| IBIS file for GS81302xxxE
| Package: standard 165pin BGA
| DQ driver is programmable
| VDD 1.8V, VDDQ 1.5V or 1.8V
| Date:
| Rev 1.1 11/12/10 1) Pin F10 on Q36 pacakge changed from DIN to PROGBUF
[IBIS Ver]   4.2
[File name]   81302xxxe.ibs
[File Rev]   1.1
[Date]   11/12/10
[Component]   GS81302D08E
[Manufacturer]   GSI Technology
[Package]
|  variable   typ   min   max
R_pkg   0.2   0.1   0.5
L_pkg   3nH   1nH   5nH
C_pkg   1.5pF   1pF   3pF
[Package Model]   81302xxxE
[Pin Mapping] pulldown_ref pullup_ref gnd_clamp_ref power_clamp_ref ext_ref
|PIN   Pull-Down   Pull-Up   Power-clamp   Gnd-clamp   EXT-ref
 A1   VSS   VDDQ   VSS   VDD
 A2   NC   NC   VSS   VDD   VREF
 A3   NC   NC   VSS   VDD   VREF
 A4   NC   NC   VSS   VDD   VREF
 A5   NC   NC   VSS   VDD   VREF
 A6   NC   NC   VSS   VDD   VREF
 A7   NC   NC   VSS   VDD   VREF
 A8   NC   NC   VSS   VDD   VREF
 A9   NC   NC   VSS   VDD   VREF
 A10   NC   NC   VSS   VDD   VREF
 A11   VSS   VDDQ   VSS   VDD
 B1   NC   NC
 B2   NC   NC
 B3   NC   NC
 B4   NC   NC   VSS   VDD   VREF
 B5   NC   NC
 B6   NC   NC   VSS   VDD   VREF
 B7   NC   NC   VSS   VDD   VREF
 B8   NC   NC   VSS   VDD   VREF
 B9   NC   NC
 B10   NC   NC
 B11   VSS   VDDQ   VSS   VDD
 C1   NC   NC
 C2   NC   NC
 C3   NC   NC
 C4   VSS   NC
 C5   NC   NC   VSS   VDD   VREF
 C6   NC   NC
 C7   NC   NC   VSS   VDD   VREF
 C8   VSS   NC
 C9   NC   NC
 C10   NC   NC
 C11   NC   NC   VSS   VDD   VREF
 D1   NC   NC
 D2   NC   NC   VSS   VDD   VREF
 D3   NC   NC
 D4   VSS   NC
 D5   VSS   NC
 D6   VSS   NC
 D7   VSS   NC
 D8   VSS   NC
 D9   NC   NC
 D10   NC   NC
 D11   NC   NC
 E1   NC   NC
 E2   NC   NC
 E3   NC   NC
 E4   NC   VDDQ
 E5   VSS   NC
 E6   VSS   NC
 E7   VSS   NC
 E8   NC   VDDQ
 E9   NC   NC
 E10   NC   NC   VSS   VDD   VREF
 E11   VSS   VDDQ   VSS   VDD
 F1   NC   NC
 F2   NC   NC
 F3   NC   NC
 F4   NC   VDDQ
 F5   NC   VDD
 F6   VSS   NC
 F7   NC   VDD
 F8   NC   VDDQ
 F9   NC   NC
 F10   NC   NC
 F11   NC   NC
 G1   NC   NC
 G2   NC   NC   VSS   VDD   VREF
 G3   VSS   VDDQ   VSS   VDD
 G4   NC   VDDQ
 G5   NC   VDD
 G6   VSS   NC
 G7   NC   VDD
 G8   NC   VDDQ
 G9   NC   NC
 G10   NC   NC
 G11   NC   NC
 H1   NC   NC   VSS   VDD   VREF
 H2   NC   VREF
 H3   NC   VDDQ
 H4   NC   VDDQ
 H5   NC   VDD
 H6   VSS   NC
 H7   NC   VDD
 H8   NC   VDDQ
 H9   NC   VDDQ
 H10   NC   VREF
 H11   NC   NC
 J1   NC   NC
 J2   NC   NC
 J3   NC   NC
 J4   NC   VDDQ
 J5   NC   VDD
 J6   VSS   NC
 J7   NC   VDD
 J8   NC   VDDQ
 J9   NC   NC
 J10   VSS   VDDQ   VSS   VDD
 J11   NC   NC   VSS   VDD   VREF
 K1   NC   NC
 K2   NC   NC
 K3   NC   NC
 K4   NC   VDDQ
 K5   NC   VDD
 K6   VSS   NC
 K7   NC   VDD
 K8   NC   VDDQ
 K9   NC   NC
 K10   NC   NC
 K11   NC   NC
 L1   NC   NC
 L2   VSS   VDDQ   VSS   VDD
 L3   NC   NC   VSS   VDD   VREF
 L4   NC   VDDQ
 L5   VSS   NC
 L6   VSS   NC
 L7   VSS   NC
 L8   NC   VDDQ
 L9   NC   NC
 L10   NC   NC
 L11   VSS   VDDQ   VSS   VDD
 M1   NC   NC
 M2   NC   NC
 M3   NC   NC
 M4   VSS   NC
 M5   VSS   NC
 M6   VSS   NC
 M7   VSS   NC
 M8   VSS   NC
 M9   NC   NC
 M10   NC   NC
 M11   NC   NC   VSS   VDD   VREF
 N1   NC   NC
 N2   NC   NC   VSS   VDD   VREF
 N3   NC   NC
 N4   VSS   NC
 N5   NC   NC   VSS   VDD   VREF
 N6   NC   NC   VSS   VDD   VREF
 N7   NC   NC   VSS   VDD   VREF
 N8   VSS   NC
 N9   NC   NC
 N10   NC   NC
 N11   NC   NC
 P1   NC   NC
 P2   NC   NC
 P3   VSS   VDDQ   VSS   VDD
 P4   NC   NC   VSS   VDD   VREF
 P5   NC   NC   VSS   VDD   VREF
 P6   NC   NC   VSS   VDD   VREF
 P7   NC   NC   VSS   VDD   VREF
 P8   NC   NC   VSS   VDD   VREF
 P9   NC   NC
 P10   NC   NC
 P11   NC   NC
 R1   VSS   VDDQ   VSS   VDD
 R2   NC   NC   VSS   VDD   VREF
 R3   NC   NC   VSS   VDD   VREF
 R4   NC   NC   VSS   VDD   VREF
 R5   NC   NC   VSS   VDD   VREF
 R6   NC   NC   VSS   VDD   VREF
 R7   NC   NC   VSS   VDD   VREF
 R8   NC   NC   VSS   VDD   VREF
 R9   NC   NC   VSS   VDD   VREF
 R10   NC   NC   VSS   VDD   VREF
 R11   NC   NC   VSS   VDD   VREF
[Pin]   signal_name model_name   R_pin   L_pin   C_pin
 A1   nCQ   ECHO   197m   2.83nH   0.820pF
 A2   SA   CONTROL   131m   1.45nH   0.544pF
 A3   SA   CONTROL   150m   1.95nH   0.604pF
 A4   nW   CONTROL   138m   1.73nH   0.628pF
 A5   nNW1   CONTROL   139m   1.69nH   0.633pF
 A6   nK   CONTROL   178m   2.50nH   0.709pF
 A7   SA   CONTROL   153m   1.96nH   0.651pF
 A8   nR   CONTROL   132m   1.54nH   0.560pF
 A9   SA   CONTROL   131m   1.40nH   0.554pF
 A10   SA   CONTROL   130m   1.44nH   0.546pF
 A11   CQ   ECHO   202m   2.94nH   0.807pF
 B1   NC   NC
 B2   NC   NC
 B3   NC   NC
 B4   SA   CONTROL   189m   2.46nH   0.773pF
 B5   NC   NC
 B6   K   CONTROL   178m   2.43nH   0.753pF
 B7   nNW0   CONTROL   159m   1.94nH   0.700pF
 B8   SA   CONTROL   164m   1.96nH   0.641pF
 B9   NC   NC
 B10   NC   NC
 B11   Q3   PROGBUF   194m   2.34nH   0.805pF
 C1   NC   NC
 C2   NC   NC
 C3   NC   NC
 C4   VSS   GND
 C5   SA   CONTROL   189m   2.60nH   0.874pF
 C6   NC   NC
 C7   SA   CONTROL   204m   2.82nH   0.820pF
 C8   VSS   GND
 C9   NC   NC
 C10   NC   NC
 C11   D3   DIN   212m   2.69nH   0.808pF
 D1   NC   NC
 D2   D4   DIN   206m   2.66nH   0.823pF
 D3   NC   NC
 D4   VSS   GND
 D5   VSS   GND
 D6   VSS   GND
 D7   VSS   GND
 D8   VSS   GND
 D9   NC   NC
 D10   NC   NC
 D11   Nc   NC
 E1   Nc   NC
 E2   Nc   NC
 E3   Q4   PROGBUF   196m   2.78nH   0.947pF
 E4   VDDQ   POWER
 E5   VSS   GND
 E6   VSS   GND
 E7   VSS   GND
 E8   VDDQ   POWER
 E9   NC   NC
 E10   D2   DIN   202m   2.76nH   0.779pF
 E11   Q2   PROGBUF   196m   2.42nH   0.803pF
 F1   NC   NC
 F2   NC   NC
 F3   NC   NC
 F4   VDDQ   POWER
 F5   VDD   POWER
 F6   VSS   GND
 F7   VDD   POWER
 F8   VDDQ   POWER
 F9   NC   NC
 F10   NC   NC
 F11   NC   NC
 G1   NC   NC
 G2   D5   DIN   210m   2.94nH   0.887pF
 G3   Q5   PROGBUF   184m   2.75nH   0.946pF
 G4   VDDQ   POWER
 G5   VDD   POWER
 G6   VSS   GND
 G7   VDD   POWER
 G8   VDDQ   POWER
 G9   NC   NC
 G10   NC   NC
 G11   NC   NC
 H1   NDoff   CONTROL   165m   1.96nH   0.637pF
 H2   VREF   POWER
 H3   VDDQ   POWER
 H4   VDDQ   POWER
 H5   VDD   POWER
 H6   VSS   GND
 H7   VDD   POWER
 H8   VDDQ   POWER
 H9   VDDQ   POWER
 H10   VREF   POWER
 H11   ZQ   NC
 J1   NC   NC
 J2   NC   NC
 J3   NC   NC
 J4   VDDQ   POWER
 J5   VDD   POWER
 J6   VSS   GND
 J7   VDD   POWER
 J8   VDDQ   POWER
 J9   NC   NC
 J10   Q1   PROGBUF   205m   2.81nH   0.844pF
 J11   D1   DIN   202m   2.51nH   0.823pF
 K1   NC   NC
 K2   NC   NC
 K3   NC   NC
 K4   VDDQ   POWER
 K5   VDD   POWER
 K6   VSS   GND
 K7   VDD   POWER
 K8   VDDQ   POWER
 K9   NC   NC
 K10   NC   NC
 K11   NC   NC
 L1   NC   NC
 L2   Q6   PROGBUF   174m   2.27nH   0.866pF
 L3   D6   DIN   185m   2.74nH   0.923pF
 L4   VDDQ   POWER
 L5   VSS   GND
 L6   VSS   GND
 L7   VSS   GND
 L8   VDDQ   POWER
 L9   NC   NC
 L10   NC   NC
 L11   Q0   PROGBUF   193m   2.31nH   0.828pF
 M1   NC   NC
 M2   NC   NC
 M3   NC   NC
 M4   VSS   GND
 M5   VSS   GND
 M6   VSS   GND
 M7   VSS   GND
 M8   VSS   GND
 M9   NC   NC
 M10   NC   NC
 M11   D0   DIN   209m   2.65nH   0.828pF
 N1   NC   NC
 N2   D7   DIN   201m   2.68nH   0.874pF
 N3   NC   NC
 N4   VSS   GND
 N5   SA   CONTROL   188m   2.45nH   0.921pF
 N6   SA   CONTROL   204m   2.83nH   0.868pF
 N7   SA   CONTROL   163m   2.11nH   0.852pF
 N8   VSS   GND
 N9   NC   NC
 N10   NC   NC
 N11   NC   NC
 P1   NC   NC
 P2   NC   NC
 P3   Q7   PROGBUF   186m   2.78nH   0.889pF
 P4   SA   CONTROL   146m   1.90nH   0.747pF
 P5   SA   CONTROL   212m   3.30nH   0.853pF
 P6   C   CONTROL   186m   2.56nH   0.853pF
 P7   SA   CONTROL   161m   2.06nH   0.701pF
 P8   SA   CONTROL   161m   2.05nH   0.660pF
 P9   NC   NC
 P10   NC   NC
 P11   NC   NC
 R1   TDO   JTAG   160m   2.03nH   0.671pF
 R2   TCK   CONTROL   166m   2.10nH   0.712pF
 R3   SA   CONTROL   153m   2.12nH   0.662pF
 R4   SA   CONTROL   180m   2.75nH   0.761pF
 R5   SA   CONTROL   176m   2.69nH   0.749pF
 R6   CBar   CONTROL   194m   3.19nH   0.788pF
 R7   SA   CONTROL   177m   2.32nH   0.736pF
 R8   SA   CONTROL   137m   1.63nH   0.576pF
 R9   SA   CONTROL   125m   1.39nH   0.547pF
 R10   TMS   CONTROL   131m   1.64nH   0.560pF
 R11   TDI   CONTROL   970m   0.91nH   0.503pF
[Component]   GS81302D09E
[Manufacturer]   GSI Technology
[Package]
|  variable   typ   min   max
R_pkg   0.2   0.1   0.5
L_pkg   3nH   1nH   5nH
C_pkg   1.5pF   1pF   3pF
[Package Model]   81302xxxE
[Pin Mapping] pulldown_ref pullup_ref gnd_clamp_ref power_clamp_ref ext_ref
|PIN   Pull-Down   Pull-Up   Power-clamp   Gnd-clamp   EXT-ref
 A1   VSS   VDDQ   VSS   VDD
 A2   NC   NC   VSS   VDD   VREF
 A3   NC   NC   VSS   VDD   VREF
 A4   NC   NC   VSS   VDD   VREF
 A5   NC   NC   VSS   VDD   VREF
 A6   NC   NC   VSS   VDD   VREF
 A7   NC   NC   VSS   VDD   VREF
 A8   NC   NC   VSS   VDD   VREF
 A9   NC   NC   VSS   VDD   VREF
 A10   NC   NC   VSS   VDD   VREF
 A11   VSS   VDDQ   VSS   VDD
 B1   NC   NC
 B2   NC   NC
 B3   NC   NC
 B4   NC   NC   VSS   VDD   VREF
 B5   NC   NC
 B6   NC   NC   VSS   VDD   VREF
 B7   NC   NC   VSS   VDD   VREF
 B8   NC   NC   VSS   VDD   VREF
 B9   NC   NC
 B10   NC   NC
 B11   VSS   VDDQ   VSS   VDD
 C1   NC   NC
 C2   NC   NC
 C3   NC   NC
 C4   VSS   NC
 C5   NC   NC   VSS   VDD   VREF
 C6   NC   NC
 C7   NC   NC   VSS   VDD   VREF
 C8   VSS   NC
 C9   NC   NC
 C10   NC   NC
 C11   NC   NC   VSS   VDD   VREF
 D1   NC   NC
 D2   NC   NC   VSS   VDD   VREF
 D3   NC   NC
 D4   VSS   NC
 D5   VSS   NC
 D6   VSS   NC
 D7   VSS   NC
 D8   VSS   NC
 D9   NC   NC
 D10   NC   NC
 D11   NC   NC
 E1   NC   NC
 E2   NC   NC
 E3   VSS   VDDQ   VSS   VDD
 E4   NC   VDDQ
 E5   VSS   NC
 E6   VSS   NC
 E7   VSS   NC
 E8   NC   VDDQ
 E9   NC   NC
 E10   NC   NC   VSS   VDD   VREF
 E11   VSS   VDDQ   VSS   VDD
 F1   NC   NC
 F2   NC   NC
 F3   NC   NC
 F4   NC   VDDQ
 F5   NC   VDD
 F6   VSS   NC
 F7   NC   VDD
 F8   NC   VDDQ
 F9   NC   NC
 F10   NC   NC
 F11   NC   NC
 G1   NC   NC
 G2   NC   NC   VSS   VDD   VREF
 G3   VSS   VDDQ   VSS   VDD
 G4   NC   VDDQ
 G5   NC   VDD
 G6   VSS   NC
 G7   NC   VDD
 G8   NC   VDDQ
 G9   NC   NC
 G10   NC   NC
 G11   NC   NC
 H1   NC   NC   VSS   VDD   VREF
 H2   NC   VREF
 H3   NC   VDDQ
 H4   NC   VDDQ
 H5   NC   VDD
 H6   VSS   NC
 H7   NC   VDD
 H8   NC   VDDQ
 H9   NC   VDDQ
 H10   NC   VREF
 H11   NC   NC
 J1   NC   NC
 J2   NC   NC
 J3   NC   NC
 J4   NC   VDDQ
 J5   NC   VDD
 J6   VSS   NC
 J7   NC   VDD
 J8   NC   VDDQ
 J9   NC   NC
 J10   VSS   VDDQ   VSS   VDD
 J11   NC   NC   VSS   VDD   VREF
 K1   NC   NC
 K2   NC   NC
 K3   NC   NC
 K4   NC   VDDQ
 K5   NC   VDD
 K6   VSS   NC
 K7   NC   VDD
 K8   NC   VDDQ
 K9   NC   NC
 K10   NC   NC
 K11   NC   NC
 L1   NC   NC
 L2   VSS   VDDQ   VSS   VDD
 L3   NC   NC   VSS   VDD   VREF
 L4   NC   VDDQ
 L5   VSS   NC
 L6   VSS   NC
 L7   VSS   NC
 L8   NC   VDDQ
 L9   NC   NC
 L10   NC   NC
 L11   VSS   VDDQ   VSS   VDD
 M1   NC   NC
 M2   NC   NC
 M3   NC   NC
 M4   VSS   NC
 M5   VSS   NC
 M6   VSS   NC
 M7   VSS   NC
 M8   VSS   NC
 M9   NC   NC
 M10   NC   NC
 M11   NC   NC   VSS   VDD   VREF
 N1   NC   NC
 N2   NC   NC   VSS   VDD   VREF
 N3   NC   NC
 N4   VSS   NC
 N5   NC   NC   VSS   VDD   VREF
 N6   NC   NC   VSS   VDD   VREF
 N7   NC   NC   VSS   VDD   VREF
 N8   VSS   NC
 N9   NC   NC
 N10   NC   NC
 N11   NC   NC
 P1   NC   NC
 P2   NC   NC
 P3   VSS   VDDQ   VSS   VDD
 P4   NC   NC   VSS   VDD   VREF
 P5   NC   NC   VSS   VDD   VREF
 P6   NC   NC   VSS   VDD   VREF
 P7   NC   NC   VSS   VDD   VREF
 P8   NC   NC   VSS   VDD   VREF
 P9   NC   NC
 P10   NC   NC   VSS   VDD   VREF
 P11   VSS   VDDQ   VSS   VDD
 R1   VSS   VDDQ   VSS   VDD
 R2   NC   NC   VSS   VDD   VREF
 R3   NC   NC   VSS   VDD   VREF
 R4   NC   NC   VSS   VDD   VREF
 R5   NC   NC   VSS   VDD   VREF
 R6   NC   NC   VSS   VDD   VREF
 R7   NC   NC   VSS   VDD   VREF
 R8   NC   NC   VSS   VDD   VREF
 R9   NC   NC   VSS   VDD   VREF
 R10   NC   NC   VSS   VDD   VREF
 R11   NC   NC   VSS   VDD   VREF
[Pin]   signal_name model_name   R_pin   L_pin   C_pin
 A1   nCQ   ECHO   197m   2.83nH   0.820pF
 A2   SA   CONTROL   131m   1.45nH   0.544pF
 A3   SA   CONTROL   150m   1.95nH   0.604pF
 A4   nW   CONTROL   138m   1.73nH   0.628pF
 A5   nBW1   CONTROL   139m   1.69nH   0.633pF
 A6   nK   CONTROL   178m   2.50nH   0.709pF
 A7   SA   CONTROL   153m   1.96nH   0.651pF
 A8   nR   CONTROL   132m   1.54nH   0.560pF
 A9   SA   CONTROL   131m   1.40nH   0.554pF
 A10   SA   CONTROL   130m   1.44nH   0.546pF
 A11   CQ   ECHO   202m   2.94nH   0.807pF
 B1   NC   NC
 B2   NC   NC
 B3   NC   NC
 B4   SA   CONTROL   189m   2.46nH   0.773pF
 B5   NC   NC
 B6   K   CONTROL   178m   2.43nH   0.753pF
 B7   NBW0   CONTROL   159m   1.94nH   0.700pF
 B8   SA   CONTROL   164m   1.96nH   0.641pF
 B9   NC   NC
 B10   NC   NC
 B11   Q4   PROGBUF   194m   2.34nH   0.805pF
 C1   NC   NC
 C2   NC   NC
 C3   NC   NC
 C4   VSS   GND
 C5   SA   CONTROL   189m   2.60nH   0.874pF
 C6   NC   NC
 C7   SA   CONTROL   204m   2.82nH   0.820pF
 C8   VSS   GND
 C9   NC   NC
 C10   NC   NC
 C11   D4   DIN   212m   2.69nH   0.808pF
 D1   NC   NC
 D2   D5   DIN   206m   2.66nH   0.823pF
 D3   NC   NC
 D4   VSS   GND
 D5   VSS   GND
 D6   VSS   GND
 D7   VSS   GND
 D8   VSS   GND
 D9   NC   NC
 D10   NC   NC
 D11   NC   NC
 E1   NC   NC
 E2   NC   NC
 E3   Q5   PROGBUF   196m   2.78nH   0.947pF
 E4   VDDQ   POWER
 E5   VSS   GND
 E6   VSS   GND
 E7   VSS   GND
 E8   VDDQ   POWER
 E9   NC   NC
 E10   D3   DIN   202m   2.76nH   0.779pF
 E11   Q3   PROGBUF   196m   2.42nH   0.803pF
 F1   NC   NC
 F2   NC   NC
 F3   NC   NC
 F4   VDDQ   POWER
 F5   VDD   POWER
 F6   VSS   GND
 F7   VDD   POWER
 F8   VDDQ   POWER
 F9   NC   NC
 F10   NC   NC
 F11   NC   NC
 G1   NC   NC
 G2   D6   DIN   210m   2.94nH   0.887pF
 G3   Q6   PROGBUF   184m   2.75nH   0.946pF
 G4   VDDQ   POWER
 G5   VDD   POWER
 G6   VSS   GND
 G7   VDD   POWER
 G8   VDDQ   POWER
 G9   NC   NC
 G10   NC   NC
 G11   NC   NC
 H1   NDoff   CONTROL   165m   1.96nH   0.637pF
 H2   VREF   POWER
 H3   VDDQ   POWER
 H4   VDDQ   POWER
 H5   VDD   POWER
 H6   VSS   GND
 H7   VDD   POWER
 H8   VDDQ   POWER
 H9   VDDQ   POWER
 H10   VREF   POWER
 H11   ZQ   NC
 J1   NC   NC
 J2   NC   NC
 J3   NC   NC
 J4   VDDQ   POWER
 J5   VDD   POWER
 J6   VSS   GND
 J7   VDD   POWER
 J8   VDDQ   POWER
 J9   NC   NC
 J10   Q2   PROGBUF   205m   2.81nH   0.844pF
 J11   D2   DIN   202m   2.51nH   0.823pF
 K1   NC   NC
 K2   NC   NC
 K3   NC   NC
 K4   VDDQ   POWER
 K5   VDD   POWER
 K6   VSS   GND
 K7   VDD   POWER
 K8   VDDQ   POWER
 K9   NC   NC
 K10   NC   NC
 K11   NC   NC
 L1   NC   NC
 L2   Q7   PROGBUF   174m   2.27nH   0.866pF
 L3   D7   DIN   185m   2.74nH   0.923pF
 L4   VDDQ   POWER
 L5   VSS   GND
 L6   VSS   GND
 L7   VSS   GND
 L8   VDDQ   POWER
 L9   NC   NC
 L10   NC   NC
 L11   Q1   PROGBUF   193m   2.31nH   0.828pF
 M1   NC   NC
 M2   NC   NC
 M3   NC   NC
 M4   VSS   GND
 M5   VSS   GND
 M6   VSS   GND
 M7   VSS   GND
 M8   VSS   GND
 M9   NC   NC
 M10   NC   NC
 M11   D1   DIN   209m   2.65nH   0.828pF
 N1   NC   NC
 N2   D8   DIN   201m   2.68nH   0.874pF
 N3   NC   NC
 N4   VSS   GND
 N5   SA   CONTROL   188m   2.45nH   0.921pF
 N6   SA   CONTROL   204m   2.83nH   0.868pF
 N7   SA   CONTROL   163m   2.11nH   0.852pF
 N8   VSS   GND
 N9   NC   NC
 N10   NC   NC
 N11   NC   NC
 P1   NC   NC
 P2   NC   NC
 P3   Q8   PROGBUF   186m   2.78nH   0.889pF
 P4   SA   CONTROL   146m   1.90nH   0.747pF
 P5   SA   CONTROL   212m   3.30nH   0.853pF
 P6   C   CONTROL   186m   2.56nH   0.853pF
 P7   SA   CONTROL   161m   2.06nH   0.701pF
 P8   SA   CONTROL   161m   2.05nH   0.660pF
 P9   NC   NC
 P10   D0   DIN   200m   2.92nH   0.813pF
 P11   Q0   PROGBUF   199m   2.52nH   0.815pF
 R1   TDO   JTAG   160m   2.03nH   0.671pF
 R2   TCK   CONTROL   166m   2.10nH   0.712pF
 R3   SA   CONTROL   153m   2.12nH   0.662pF
 R4   SA   CONTROL   180m   2.75nH   0.761pF
 R5   SA   CONTROL   176m   2.69nH   0.749pF
 R6   CBar   CONTROL   194m   3.19nH   0.788pF
 R7   SA   CONTROL   177m   2.32nH   0.736pF
 R8   SA   CONTROL   137m   1.63nH   0.576pF
 R9   SA   CONTROL   125m   1.39nH   0.547pF
 R10   TMS   CONTROL   131m   1.64nH   0.560pF
 R11   TDI   CONTROL   970m   0.91nH   0.503pF
[Component]   GS81302D18E
[Manufacturer]   GSI Technology
[Package]
|  variable   typ   min   max
R_pkg   0.2   0.1   0.5
L_pkg   3nH   1nH   5nH
C_pkg   1.5pF   1pF   3pF
[Package Model]   81302xxxE
[Pin Mapping] pulldown_ref pullup_ref gnd_clamp_ref power_clamp_ref ext_ref
|PIN   Pull-Down   Pull-Up   Power-clamp   Gnd-clamp   EXT-ref
 A1   VSS   VDDQ   VSS   VDD
 A2   NC   NC   VSS   VDD   VREF
 A3   NC   NC   VSS   VDD   VREF
 A4   NC   NC   VSS   VDD   VREF
 A5   NC   NC   VSS   VDD   VREF
 A6   NC   NC   VSS   VDD   VREF
 A7   NC   NC
 A8   NC   NC   VSS   VDD   VREF
 A9   NC   NC   VSS   VDD   VREF
 A10   NC   NC   VSS   VDD   VREF
 A11   VSS   VDDQ   VSS   VDD
 B1   NC   NC
 B2   VSS   VDDQ   VSS   VDD
 B3   NC   NC   VSS   VDD   VREF
 B4   NC   NC   VSS   VDD   VREF
 B5   NC   NC
 B6   NC   NC   VSS   VDD   VREF
 B7   NC   NC   VSS   VDD   VREF
 B8   NC   NC   VSS   VDD   VREF
 B9   NC   NC
 B10   NC   NC
 B11   VSS   VDDQ   VSS   VDD
 C1   NC   NC
 C2   NC   NC
 C3   NC   NC   VSS   VDD   VREF
 C4   VSS   NC
 C5   NC   NC   VSS   VDD   VREF
 C6   NC   NC
 C7   NC   NC   VSS   VDD   VREF
 C8   VSS   NC
 C9   NC   NC
 C10   VSS   VDDQ   VSS   VDD
 C11   NC   NC   VSS   VDD   VREF
 D1   NC   NC
 D2   NC   NC   VSS   VDD   VREF
 D3   VSS   VDDQ   VSS   VDD
 D4   VSS   NC
 D5   VSS   NC
 D6   VSS   NC
 D7   VSS   NC
 D8   VSS   NC
 D9   NC   NC
 D10   NC   NC
 D11   NC   NC   VSS   VDD   VREF
 E1   NC   NC
 E2   NC   NC
 E3   VSS   VDDQ   VSS   VDD
 E4   NC   VDDQ
 E5   VSS   NC
 E6   VSS   NC
 E7   VSS   NC
 E8   NC   VDDQ
 E9   NC   NC
 E10   NC   NC   VSS   VDD   VREF
 E11   VSS   VDDQ   VSS   VDD
 F1   NC   NC
 F2   VSS   VDDQ   VSS   VDD
 F3   NC   NC   VSS   VDD   VREF
 F4   NC   VDDQ
 F5   NC   VDD
 F6   VSS   NC
 F7   NC   VDD
 F8   NC   VDDQ
 F9   NC   NC
 F10   NC   NC
 F11   VSS   VDDQ   VSS   VDD
 G1   NC   NC
 G2   NC   NC   VSS   VDD   VREF
 G3   VSS   VDDQ   VSS   VDD
 G4   NC   VDDQ
 G5   NC   VDD
 G6   VSS   NC
 G7   NC   VDD
 G8   NC   VDDQ
 G9   NC   NC
 G10   NC   NC
 G11   NC   NC   VSS   VDD   VREF
 H1   NC   NC   VSS   VDD   VREF
 H2   NC   VREF
 H3   NC   VDDQ
 H4   NC   VDDQ
 H5   NC   VDD
 H6   VSS   NC
 H7   NC   VDD
 H8   NC   VDDQ
 H9   NC   VDDQ
 H10   NC   VREF
 H11   NC   NC
 J1   NC   NC
 J2   NC   NC
 J3   NC   NC   VSS   VDD   VREF
 J4   NC   VDDQ
 J5   NC   VDD
 J6   VSS   NC
 J7   NC   VDD
 J8   NC   VDDQ
 J9   NC   NC
 J10   VSS   VDDQ   VSS   VDD
 J11   NC   NC   VSS   VDD   VREF
 K1   NC   NC
 K2   NC   NC
 K3   VSS   VDDQ   VSS   VDD
 K4   NC   VDDQ
 K5   NC   VDD
 K6   VSS   NC
 K7   NC   VDD
 K8   NC   VDDQ
 K9   NC   NC
 K10   NC   NC   VSS   VDD   VREF
 K11   VSS   VDDQ   VSS   VDD
 L1   NC   NC
 L2   VSS   VDDQ   VSS   VDD
 L3   NC   NC   VSS   VDD   VREF
 L4   NC   VDDQ
 L5   VSS   NC
 L6   VSS   NC
 L7   VSS   NC
 L8   NC   VDDQ
 L9   NC   NC
 L10   NC   NC
 L11   VSS   VDDQ   VSS   VDD
 M1   NC   NC
 M2   NC   NC
 M3   NC   NC   VSS   VDD   VREF
 M4   VSS   NC
 M5   VSS   NC
 M6   VSS   NC
 M7   VSS   NC
 M8   VSS   NC
 M9   NC   NC
 M10   VSS   VDDQ   VSS   VDD
 M11   NC   NC   VSS   VDD   VREF
 N1   NC   NC
 N2   NC   NC   VSS   VDD   VREF
 N3   VSS   VDDQ   VSS   VDD
 N4   VSS   NC
 N5   NC   NC   VSS   VDD   VREF
 N6   NC   NC   VSS   VDD   VREF
 N7   NC   NC   VSS   VDD   VREF
 N8   VSS   NC
 N9   NC   NC
 N10   NC   NC
 N11   NC   NC   VSS   VDD   VREF
 P1   NC   NC
 P2   NC   NC
 P3   VSS   VDDQ   VSS   VDD
 P4   NC   NC   VSS   VDD   VREF
 P5   NC   NC   VSS   VDD   VREF
 P6   NC   NC   VSS   VDD   VREF
 P7   NC   NC   VSS   VDD   VREF
 P8   NC   NC   VSS   VDD   VREF
 P9   NC   NC
 P10   NC   NC   VSS   VDD   VREF
 P11   VSS   VDDQ   VSS   VDD
 R1   VSS   VDDQ   VSS   VDD
 R2   NC   NC   VSS   VDD   VREF
 R3   NC   NC   VSS   VDD   VREF
 R4   NC   NC   VSS   VDD   VREF
 R5   NC   NC   VSS   VDD   VREF
 R6   NC   NC   VSS   VDD   VREF
 R7   NC   NC   VSS   VDD   VREF
 R8   NC   NC   VSS   VDD   VREF
 R9   NC   NC   VSS   VDD   VREF
 R10   NC   NC   VSS   VDD   VREF
 R11   NC   NC   VSS   VDD   VREF
[Pin]   signal_name model_name   R_pin   L_pin   C_pin
 A1   nCQ   ECHO   197m   2.83nH   0.820pF
 A2   SA   CONTROL   131m   1.45nH   0.544pF
 A3   SA   CONTROL   150m   1.95nH   0.604pF
 A4   nW   CONTROL   138m   1.73nH   0.628pF
 A5   nBW1   CONTROL   139m   1.69nH   0.633pF
 A6   nK   CONTROL   178m   2.50nH   0.709pF
 A7   NC   NC
 A8   nR   CONTROL   132m   1.54nH   0.560pF
 A9   SA   CONTROL   131m   1.40nH   0.554pF
 A10   SA   CONTROL   130m   1.44nH   0.546pF
 A11   CQ   ECHO   202m   2.94nH   0.807pF
 B1   NC   NC
 B2   Q9   PROGBUF   208m   2.60nH   0.845pF
 B3   D9   DIN   225m   2.97nH   0.904pF
 B4   SA   CONTROL   189m   2.46nH   0.773pF
 B5   NC   NC
 B6   K   CONTROL   178m   2.43nH   0.753pF
 B7   NBW0   CONTROL   159m   1.94nH   0.700pF
 B8   SA   CONTROL   164m   1.96nH   0.641pF
 B9   NC   NC
 B10   NC   NC
 B11   Q8   PROGBUF   194m   2.34nH   0.805pF
 C1   NC   NC
 C2   NC   NC
 C3   D10   DIN   220m   3.32nH   0.901pF
 C4   VSS   GND
 C5   SA   CONTROL   189m   2.60nH   0.874pF
 C6   NC   NC
 C7   SA   CONTROL   204m   2.82nH   0.820pF
 C8   VSS   GND
 C9   NC   NC
 C10   Q7   PROGBUF   215m   3.12nH   0.809pF
 C11   D8   DIN   212m   2.69nH   0.808pF
 D1   NC   NC
 D2   D11   DIN   206m   2.66nH   0.823pF
 D3   Q10   PROGBUF   189m   2.60nH   0.910pF
 D4   VSS   GND
 D5   VSS   GND
 D6   VSS   GND
 D7   VSS   GND
 D8   VSS   GND
 D9   NC   NC
 D10   NC   NC
 D11   D7   DIN   192m   2.41nH   0.793pF
 E1   NC   NC
 E2   NC   NC
 E3   Q11   PROGBUF   196m   2.78nH   0.947pF
 E4   VDDQ   POWER
 E5   VSS   GND
 E6   VSS   GND
 E7   VSS   GND
 E8   VDDQ   POWER
 E9   NC   NC
 E10   D6   DIN   202m   2.76nH   0.779pF
 E11   Q6   PROGBUF   196m   2.42nH   0.803pF
 F1   NC   NC
 F2   Q12   PROGBUF   211m   2.71nH   0.850pF
 F3   D12   DIN   184m   2.63nH   0.913pF
 F4   VDDQ   POWER
 F5   VDD   POWER
 F6   VSS   GND
 F7   VDD   POWER
 F8   VDDQ   POWER
 F9   NC   NC
 F10   NC   NC
 F11   Q5   PROGBUF   192m   2.33nH   0.795pF
 G1   NC   NC
 G2   D13   DIN   210m   2.94nH   0.887pF
 G3   Q13   PROGBUF   184m   2.75nH   0.946pF
 G4   VDDQ   POWER
 G5   VDD   POWER
 G6   VSS   GND
 G7   VDD   POWER
 G8   VDDQ   POWER
 G9   NC   NC
 G10   NC   NC
 G11   D5   DIN   207m   2.66nH   0.842pF
 H1   NDoff   CONTROL   165m   1.96nH   0.637pF
 H2   VREF   POWER
 H3   VDDQ   POWER
 H4   VDDQ   POWER
 H5   VDD   POWER
 H6   VSS   GND
 H7   VDD   POWER
 H8   VDDQ   POWER
 H9   VDDQ   POWER
 H10   VREF   POWER
 H11   ZQ   NC
 J1   NC   NC
 J2   NC   NC
 J3   D14   DIN   226m   3.23nH   0.948pF
 J4   VDDQ   POWER
 J5   VDD   POWER
 J6   VSS   GND
 J7   VDD   POWER
 J8   VDDQ   POWER
 J9   NC   NC
 J10   Q4   PROGBUF   205m   2.81nH   0.844pF
 J11   D4   DIN   202m   2.51nH   0.823pF
 K1   NC   NC
 K2   NC   NC
 K3   Q14   PROGBUF   189m   2.85nH   0.951pF
 K4   VDDQ   POWER
 K5   VDD   POWER
 K6   VSS   GND
 K7   VDD   POWER
 K8   VDDQ   POWER
 K9   NC   NC
 K10   D3   DIN   202m   2.80nH   0.834pF
 K11   Q3   PROGBUF   192m   2.33nH   0.811pF
 L1   NC   NC
 L2   Q15   PROGBUF   174m   2.27nH   0.866pF
 L3   D15   DIN   185m   2.74nH   0.923pF
 L4   VDDQ   POWER
 L5   VSS   GND
 L6   VSS   GND
 L7   VSS   GND
 L8   VDDQ   POWER
 L9   NC   NC
 L10   NC   NC
 L11   Q2   PROGBUF   193m   2.31nH   0.828pF
 M1   NC   NC
 M2   NC   NC
 M3   D16   DIN   227m   3.44nH   0.929pF
 M4   VSS   GND
 M5   VSS   GND
 M6   VSS   GND
 M7   VSS   GND
 M8   VSS   GND
 M9   NC   NC
 M10   Q1   PROGBUF   208m   3.05nH   0.827pF
 M11   D2   DIN   209m   2.65nH   0.828pF
 N1   NC   NC
 N2   D17   DIN   201m   2.68nH   0.874pF
 N3   Q16   PROGBUF   186m   2.86nH   0.943pF
 N4   VSS   GND
 N5   SA   CONTROL   188m   2.45nH   0.921pF
 N6   SA   CONTROL   204m   2.83nH   0.868pF
 N7   SA   CONTROL   163m   2.11nH   0.852pF
 N8   VSS   GND
 N9   NC   NC
 N10   NC   NC
 N11   D1   DIN   190m   2.33nH   0.805pF
 P1   NC   NC
 P2   NC   NC
 P3   Q17   PROGBUF   186m   2.78nH   0.889pF
 P4   SA   CONTROL   146m   1.90nH   0.747pF
 P5   SA   CONTROL   212m   3.30nH   0.853pF
 P6   C   CONTROL   186m   2.56nH   0.853pF
 P7   SA   CONTROL   161m   2.06nH   0.701pF
 P8   SA   CONTROL   161m   2.05nH   0.660pF
 P9   NC   NC
 P10   D0   DIN   200m   2.92nH   0.813pF
 P11   Q0   PROGBUF   199m   2.52nH   0.815pF
 R1   TDO   JTAG   160m   2.03nH   0.671pF
 R2   TCK   CONTROL   166m   2.10nH   0.712pF
 R3   SA   CONTROL   153m   2.12nH   0.662pF
 R4   SA   CONTROL   180m   2.75nH   0.761pF
 R5   SA   CONTROL   176m   2.69nH   0.749pF
 R6   CBar   CONTROL   194m   3.19nH   0.788pF
 R7   SA   CONTROL   177m   2.32nH   0.736pF
 R8   SA   CONTROL   137m   1.63nH   0.576pF
 R9   SA   CONTROL   125m   1.39nH   0.547pF
 R10   TMS   CONTROL   131m   1.64nH   0.560pF
 R11   TDI   CONTROL   970m   0.91nH   0.503pF
[Component]   GS81302D19E
[Manufacturer]   GSI Technology
[Package]
|  variable   typ   min   max
R_pkg   0.2   0.1   0.5
L_pkg   3nH   1nH   5nH
C_pkg   1.5pF   1pF   3pF
[Package Model]   81302xxxE
[Pin Mapping] pulldown_ref pullup_ref gnd_clamp_ref power_clamp_ref ext_ref
|PIN   Pull-Down   Pull-Up   Power-clamp   Gnd-clamp   EXT-ref
 A1   VSS   VDDQ   VSS   VDD
 A2   NC   NC   VSS   VDD   VREF
 A3   NC   NC   VSS   VDD   VREF
 A4   NC   NC   VSS   VDD   VREF
 A5   NC   NC   VSS   VDD   VREF
 A6   NC   NC   VSS   VDD   VREF
 A7   NC   NC
 A8   NC   NC   VSS   VDD   VREF
 A9   NC   NC   VSS   VDD   VREF
 A10   NC   NC   VSS   VDD   VREF
 A11   VSS   VDDQ   VSS   VDD
 B1   NC   NC
 B2   VSS   VDDQ   VSS   VDD
 B3   NC   NC   VSS   VDD   VREF
 B4   NC   NC   VSS   VDD   VREF
 B5   NC   NC
 B6   NC   NC   VSS   VDD   VREF
 B7   NC   NC   VSS   VDD   VREF
 B8   NC   NC   VSS   VDD   VREF
 B9   NC   NC
 B10   NC   NC
 B11   VSS   VDDQ   VSS   VDD
 C1   NC   NC
 C2   NC   NC
 C3   NC   NC   VSS   VDD   VREF
 C4   VSS   NC
 C5   NC   NC   VSS   VDD   VREF
 C6   NC   NC
 C7   NC   NC   VSS   VDD   VREF
 C8   VSS   NC
 C9   NC   NC
 C10   VSS   VDDQ   VSS   VDD
 C11   NC   NC   VSS   VDD   VREF
 D1   NC   NC
 D2   NC   NC   VSS   VDD   VREF
 D3   VSS   VDDQ   VSS   VDD
 D4   VSS   NC
 D5   VSS   NC
 D6   VSS   NC
 D7   VSS   NC
 D8   VSS   NC
 D9   NC   NC
 D10   NC   NC
 D11   NC   NC   VSS   VDD   VREF
 E1   NC   NC
 E2   NC   NC
 E3   VSS   VDDQ   VSS   VDD
 E4   NC   VDDQ
 E5   VSS   NC
 E6   VSS   NC
 E7   VSS   NC
 E8   NC   VDDQ
 E9   NC   NC
 E10   NC   NC   VSS   VDD   VREF
 E11   VSS   VDDQ   VSS   VDD
 F1   NC   NC
 F2   VSS   VDDQ   VSS   VDD
 F3   NC   NC   VSS   VDD   VREF
 F4   NC   VDDQ
 F5   NC   VDD
 F6   VSS   NC
 F7   NC   VDD
 F8   NC   VDDQ
 F9   NC   NC
 F10   NC   NC
 F11   VSS   VDDQ   VSS   VDD
 G1   NC   NC
 G2   NC   NC   VSS   VDD   VREF
 G3   VSS   VDDQ   VSS   VDD
 G4   NC   VDDQ
 G5   NC   VDD
 G6   VSS   NC
 G7   NC   VDD
 G8   NC   VDDQ
 G9   NC   NC
 G10   NC   NC
 G11   NC   NC   VSS   VDD   VREF
 H1   NC   NC   VSS   VDD   VREF
 H2   NC   VREF
 H3   NC   VDDQ
 H4   NC   VDDQ
 H5   NC   VDD
 H6   VSS   NC
 H7   NC   VDD
 H8   NC   VDDQ
 H9   NC   VDDQ
 H10   NC   VREF
 H11   NC   NC
 J1   NC   NC
 J2   NC   NC
 J3   NC   NC   VSS   VDD   VREF
 J4   NC   VDDQ
 J5   NC   VDD
 J6   VSS   NC
 J7   NC   VDD
 J8   NC   VDDQ
 J9   NC   NC
 J10   VSS   VDDQ   VSS   VDD
 J11   NC   NC   VSS   VDD   VREF
 K1   NC   NC
 K2   NC   NC
 K3   VSS   VDDQ   VSS   VDD
 K4   NC   VDDQ
 K5   NC   VDD
 K6   VSS   NC
 K7   NC   VDD
 K8   NC   VDDQ
 K9   NC   NC
 K10   NC   NC   VSS   VDD   VREF
 K11   VSS   VDDQ   VSS   VDD
 L1   NC   NC
 L2   VSS   VDDQ   VSS   VDD
 L3   NC   NC   VSS   VDD   VREF
 L4   NC   VDDQ
 L5   VSS   NC
 L6   VSS   NC
 L7   VSS   NC
 L8   NC   VDDQ
 L9   NC   NC
 L10   NC   NC
 L11   VSS   VDDQ   VSS   VDD
 M1   NC   NC
 M2   NC   NC
 M3   NC   NC   VSS   VDD   VREF
 M4   VSS   NC
 M5   VSS   NC
 M6   VSS   NC
 M7   VSS   NC
 M8   VSS   NC
 M9   NC   NC
 M10   VSS   VDDQ   VSS   VDD
 M11   NC   NC   VSS   VDD   VREF
 N1   NC   NC
 N2   NC   NC   VSS   VDD   VREF
 N3   VSS   VDDQ   VSS   VDD
 N4   VSS   NC
 N5   NC   NC   VSS   VDD   VREF
 N6   NC   NC   VSS   VDD   VREF
 N7   NC   NC   VSS   VDD   VREF
 N8   VSS   NC
 N9   NC   NC
 N10   NC   NC
 N11   NC   NC   VSS   VDD   VREF
 P1   NC   NC
 P2   NC   NC
 P3   VSS   VDDQ   VSS   VDD
 P4   NC   NC   VSS   VDD   VREF
 P5   NC   NC   VSS   VDD   VREF
 P6   VSS   VDDQ   VSS   VDD
 P7   NC   NC   VSS   VDD   VREF
 P8   NC   NC   VSS   VDD   VREF
 P9   NC   NC
 P10   NC   NC   VSS   VDD   VREF
 P11   VSS   VDDQ   VSS   VDD
 R1   VSS   VDDQ   VSS   VDD
 R2   NC   NC   VSS   VDD   VREF
 R3   NC   NC   VSS   VDD   VREF
 R4   NC   NC   VSS   VDD   VREF
 R5   NC   NC   VSS   VDD   VREF
 R6   NC   NC
 R7   NC   NC   VSS   VDD   VREF
 R8   NC   NC   VSS   VDD   VREF
 R9   NC   NC   VSS   VDD   VREF
 R10   NC   NC   VSS   VDD   VREF
 R11   NC   NC   VSS   VDD   VREF
[Pin]   signal_name model_name   R_pin   L_pin   C_pin
 A1   nCQ   ECHO   197m   2.83nH   0.820pF
 A2   SA   CONTROL   131m   1.45nH   0.544pF
 A3   SA   CONTROL   150m   1.95nH   0.604pF
 A4   nW   CONTROL   138m   1.73nH   0.628pF
 A5   nBW1   CONTROL   139m   1.69nH   0.633pF
 A6   nK   CONTROL   178m   2.50nH   0.709pF
 A7   NC   NC
 A8   nR   CONTROL   132m   1.54nH   0.560pF
 A9   SA   CONTROL   131m   1.40nH   0.554pF
 A10   SA   CONTROL   130m   1.44nH   0.546pF
 A11   CQ   ECHO   202m   2.94nH   0.807pF
 B1   NC   NC
 B2   Q9   PROGBUF   208m   2.60nH   0.845pF
 B3   D9   DIN   225m   2.97nH   0.904pF
 B4   SA   CONTROL   189m   2.46nH   0.773pF
 B5   NC   NC
 B6   K   CONTROL   178m   2.43nH   0.753pF
 B7   NBW0   CONTROL   159m   1.94nH   0.700pF
 B8   SA   CONTROL   164m   1.96nH   0.641pF
 B9   NC   NC
 B10   NC   NC
 B11   Q8   PROGBUF   194m   2.34nH   0.805pF
 C1   NC   NC
 C2   NC   NC
 C3   D10   DIN   220m   3.32nH   0.901pF
 C4   VSS   GND
 C5   SA   CONTROL   189m   2.60nH   0.874pF
 C6   NC   NC
 C7   SA   CONTROL   204m   2.82nH   0.820pF
 C8   VSS   GND
 C9   NC   NC
 C10   Q7   PROGBUF   215m   3.12nH   0.809pF
 C11   D8   DIN   212m   2.69nH   0.808pF
 D1   NC   NC
 D2   D11   DIN   206m   2.66nH   0.823pF
 D3   Q10   PROGBUF   189m   2.60nH   0.910pF
 D4   VSS   GND
 D5   VSS   GND
 D6   VSS   GND
 D7   VSS   GND
 D8   VSS   GND
 D9   NC   NC
 D10   NC   NC
 D11   D7   DIN   192m   2.41nH   0.793pF
 E1   NC   NC
 E2   NC   NC
 E3   Q11   PROGBUF   196m   2.78nH   0.947pF
 E4   VDDQ   POWER
 E5   VSS   GND
 E6   VSS   GND
 E7   VSS   GND
 E8   VDDQ   POWER
 E9   NC   NC
 E10   D6   DIN   202m   2.76nH   0.779pF
 E11   Q6   PROGBUF   196m   2.42nH   0.803pF
 F1   NC   NC
 F2   Q12   PROGBUF   211m   2.71nH   0.850pF
 F3   D12   DIN   184m   2.63nH   0.913pF
 F4   VDDQ   POWER
 F5   VDD   POWER
 F6   VSS   GND
 F7   VDD   POWER
 F8   VDDQ   POWER
 F9   NC   NC
 F10   NC   NC
 F11   Q5   PROGBUF   192m   2.33nH   0.795pF
 G1   NC   NC
 G2   D13   DIN   210m   2.94nH   0.887pF
 G3   Q13   PROGBUF   184m   2.75nH   0.946pF
 G4   VDDQ   POWER
 G5   VDD   POWER
 G6   VSS   GND
 G7   VDD   POWER
 G8   VDDQ   POWER
 G9   NC   NC
 G10   NC   NC
 G11   D5   DIN   207m   2.66nH   0.842pF
 H1   NDoff   CONTROL   165m   1.96nH   0.637pF
 H2   VREF   POWER
 H3   VDDQ   POWER
 H4   VDDQ   POWER
 H5   VDD   POWER
 H6   VSS   GND
 H7   VDD   POWER
 H8   VDDQ   POWER
 H9   VDDQ   POWER
 H10   VREF   POWER
 H11   ZQ   NC
 J1   NC   NC
 J2   NC   NC
 J3   D14   DIN   226m   3.23nH   0.948pF
 J4   VDDQ   POWER
 J5   VDD   POWER
 J6   VSS   GND
 J7   VDD   POWER
 J8   VDDQ   POWER
 J9   NC   NC
 J10   Q4   PROGBUF   205m   2.81nH   0.844pF
 J11   D4   DIN   202m   2.51nH   0.823pF
 K1   NC   NC
 K2   NC   NC
 K3   Q14   PROGBUF   189m   2.85nH   0.951pF
 K4   VDDQ   POWER
 K5   VDD   POWER
 K6   VSS   GND
 K7   VDD   POWER
 K8   VDDQ   POWER
 K9   NC   NC
 K10   D3   DIN   202m   2.80nH   0.834pF
 K11   Q3   PROGBUF   192m   2.33nH   0.811pF
 L1   NC   NC
 L2   Q15   PROGBUF   174m   2.27nH   0.866pF
 L3   D15   DIN   185m   2.74nH   0.923pF
 L4   VDDQ   POWER
 L5   VSS   GND
 L6   VSS   GND
 L7   VSS   GND
 L8   VDDQ   POWER
 L9   NC   NC
 L10   NC   NC
 L11   Q2   PROGBUF   193m   2.31nH   0.828pF
 M1   NC   NC
 M2   NC   NC
 M3   D16   DIN   227m   3.44nH   0.929pF
 M4   VSS   GND
 M5   VSS   GND
 M6   VSS   GND
 M7   VSS   GND
 M8   VSS   GND
 M9   NC   NC
 M10   Q1   PROGBUF   208m   3.05nH   0.827pF
 M11   D2   DIN   209m   2.65nH   0.828pF
 N1   NC   NC
 N2   D17   DIN   201m   2.68nH   0.874pF
 N3   Q16   PROGBUF   186m   2.86nH   0.943pF
 N4   VSS   GND
 N5   SA   CONTROL   188m   2.45nH   0.921pF
 N6   SA   CONTROL   204m   2.83nH   0.868pF
 N7   SA   CONTROL   163m   2.11nH   0.852pF
 N8   VSS   GND
 N9   NC   NC
 N10   NC   NC
 N11   D1   DIN   190m   2.33nH   0.805pF
 P1   NC   NC
 P2   NC   NC
 P3   Q17   PROGBUF   186m   2.78nH   0.889pF
 P4   SA   CONTROL   146m   1.90nH   0.747pF
 P5   SA   CONTROL   212m   3.30nH   0.853pF
 P6   QVLD   ECHO   186m   2.56nH   0.853pF
 P7   SA   CONTROL   161m   2.06nH   0.701pF
 P8   SA   CONTROL   161m   2.05nH   0.660pF
 P9   NC   NC
 P10   D0   DIN   200m   2.92nH   0.813pF
 P11   Q0   PROGBUF   199m   2.52nH   0.815pF
 R1   TDO   JTAG   160m   2.03nH   0.671pF
 R2   TCK   CONTROL   166m   2.10nH   0.712pF
 R3   SA   CONTROL   153m   2.12nH   0.662pF
 R4   SA   CONTROL   180m   2.75nH   0.761pF
 R5   SA   CONTROL   176m   2.69nH   0.749pF
 R6   NC   NC
 R7   SA   CONTROL   177m   2.32nH   0.736pF
 R8   SA   CONTROL   137m   1.63nH   0.576pF
 R9   SA   CONTROL   125m   1.39nH   0.547pF
 R10   TMS   CONTROL   131m   1.64nH   0.560pF
 R11   TDI   CONTROL   970m   0.91nH   0.503pF
[Component]   GS81302D20E
[Manufacturer]   GSI Technology
[Package]
|  variable   typ   min   max
R_pkg   0.2   0.1   0.5
L_pkg   3nH   1nH   5nH
C_pkg   1.5pF   1pF   3pF
[Package Model]   81302xxxE
[Pin Mapping] pulldown_ref pullup_ref gnd_clamp_ref power_clamp_ref ext_ref
|PIN   Pull-Down   Pull-Up   Power-clamp   Gnd-clamp   EXT-ref
 A1   VSS   VDDQ   VSS   VDD
 A2   NC   NC   VSS   VDD   VREF
 A3   NC   NC   VSS   VDD   VREF
 A4   NC   NC   VSS   VDD   VREF
 A5   NC   NC   VSS   VDD   VREF
 A6   NC   NC   VSS   VDD   VREF
 A7   NC   NC
 A8   NC   NC   VSS   VDD   VREF
 A9   NC   NC   VSS   VDD   VREF
 A10   NC   NC   VSS   VDD   VREF
 A11   VSS   VDDQ   VSS   VDD
 B1   NC   NC
 B2   VSS   VDDQ   VSS   VDD
 B3   NC   NC   VSS   VDD   VREF
 B4   NC   NC   VSS   VDD   VREF
 B5   NC   NC
 B6   NC   NC   VSS   VDD   VREF
 B7   NC   NC   VSS   VDD   VREF
 B8   NC   NC   VSS   VDD   VREF
 B9   NC   NC
 B10   NC   NC
 B11   VSS   VDDQ   VSS   VDD
 C1   NC   NC
 C2   NC   NC
 C3   NC   NC   VSS   VDD   VREF
 C4   VSS   NC
 C5   NC   NC   VSS   VDD   VREF
 C6   NC   NC
 C7   NC   NC   VSS   VDD   VREF
 C8   VSS   NC
 C9   NC   NC
 C10   VSS   VDDQ   VSS   VDD
 C11   NC   NC   VSS   VDD   VREF
 D1   NC   NC
 D2   NC   NC   VSS   VDD   VREF
 D3   VSS   VDDQ   VSS   VDD
 D4   VSS   NC
 D5   VSS   NC
 D6   VSS   NC
 D7   VSS   NC
 D8   VSS   NC
 D9   NC   NC
 D10   NC   NC
 D11   NC   NC   VSS   VDD   VREF
 E1   NC   NC
 E2   NC   NC
 E3   VSS   VDDQ   VSS   VDD
 E4   NC   VDDQ
 E5   VSS   NC
 E6   VSS   NC
 E7   VSS   NC
 E8   NC   VDDQ
 E9   NC   NC
 E10   NC   NC   VSS   VDD   VREF
 E11   VSS   VDDQ   VSS   VDD
 F1   NC   NC
 F2   VSS   VDDQ   VSS   VDD
 F3   NC   NC   VSS   VDD   VREF
 F4   NC   VDDQ
 F5   NC   VDD
 F6   VSS   NC
 F7   NC   VDD
 F8   NC   VDDQ
 F9   NC   NC
 F10   NC   NC
 F11   VSS   VDDQ   VSS   VDD
 G1   NC   NC
 G2   NC   NC   VSS   VDD   VREF
 G3   VSS   VDDQ   VSS   VDD
 G4   NC   VDDQ
 G5   NC   VDD
 G6   VSS   NC
 G7   NC   VDD
 G8   NC   VDDQ
 G9   NC   NC
 G10   NC   NC
 G11   NC   NC   VSS   VDD   VREF
 H1   NC   NC   VSS   VDD   VREF
 H2   NC   VREF
 H3   NC   VDDQ
 H4   NC   VDDQ
 H5   NC   VDD
 H6   VSS   NC
 H7   NC   VDD
 H8   NC   VDDQ
 H9   NC   VDDQ
 H10   NC   VREF
 H11   NC   NC
 J1   NC   NC
 J2   NC   NC
 J3   NC   NC   VSS   VDD   VREF
 J4   NC   VDDQ
 J5   NC   VDD
 J6   VSS   NC
 J7   NC   VDD
 J8   NC   VDDQ
 J9   NC   NC
 J10   VSS   VDDQ   VSS   VDD
 J11   NC   NC   VSS   VDD   VREF
 K1   NC   NC
 K2   NC   NC
 K3   VSS   VDDQ   VSS   VDD
 K4   NC   VDDQ
 K5   NC   VDD
 K6   VSS   NC
 K7   NC   VDD
 K8   NC   VDDQ
 K9   NC   NC
 K10   NC   NC   VSS   VDD   VREF
 K11   VSS   VDDQ   VSS   VDD
 L1   NC   NC
 L2   VSS   VDDQ   VSS   VDD
 L3   NC   NC   VSS   VDD   VREF
 L4   NC   VDDQ
 L5   VSS   NC
 L6   VSS   NC
 L7   VSS   NC
 L8   NC   VDDQ
 L9   NC   NC
 L10   NC   NC
 L11   VSS   VDDQ   VSS   VDD
 M1   NC   NC
 M2   NC   NC
 M3   NC   NC   VSS   VDD   VREF
 M4   VSS   NC
 M5   VSS   NC
 M6   VSS   NC
 M7   VSS   NC
 M8   VSS   NC
 M9   NC   NC
 M10   VSS   VDDQ   VSS   VDD
 M11   NC   NC   VSS   VDD   VREF
 N1   NC   NC
 N2   NC   NC   VSS   VDD   VREF
 N3   VSS   VDDQ   VSS   VDD
 N4   VSS   NC
 N5   NC   NC   VSS   VDD   VREF
 N6   NC   NC   VSS   VDD   VREF
 N7   NC   NC   VSS   VDD   VREF
 N8   VSS   NC
 N9   NC   NC
 N10   NC   NC
 N11   NC   NC   VSS   VDD   VREF
 P1   NC   NC
 P2   NC   NC
 P3   VSS   VDDQ   VSS   VDD
 P4   NC   NC   VSS   VDD   VREF
 P5   NC   NC   VSS   VDD   VREF
 P6   VSS   VDDQ   VSS   VDD
 P7   NC   NC   VSS   VDD   VREF
 P8   NC   NC   VSS   VDD   VREF
 P9   NC   NC
 P10   NC   NC   VSS   VDD   VREF
 P11   VSS   VDDQ   VSS   VDD
 R1   VSS   VDDQ   VSS   VDD
 R2   NC   NC   VSS   VDD   VREF
 R3   NC   NC   VSS   VDD   VREF
 R4   NC   NC   VSS   VDD   VREF
 R5   NC   NC   VSS   VDD   VREF
 R6   NC   NC
 R7   NC   NC   VSS   VDD   VREF
 R8   NC   NC   VSS   VDD   VREF
 R9   NC   NC   VSS   VDD   VREF
 R10   NC   NC   VSS   VDD   VREF
 R11   NC   NC   VSS   VDD   VREF
[Pin]   signal_name model_name   R_pin   L_pin   C_pin
 A1   nCQ   ECHO   197m   2.83nH   0.820pF
 A2   SA   CONTROL   131m   1.45nH   0.544pF
 A3   SA   CONTROL   150m   1.95nH   0.604pF
 A4   nW   CONTROL   138m   1.73nH   0.628pF
 A5   nBW1   CONTROL   139m   1.69nH   0.633pF
 A6   nK   CONTROL   178m   2.50nH   0.709pF
 A7   NC   NC
 A8   nR   CONTROL   132m   1.54nH   0.560pF
 A9   SA   CONTROL   131m   1.40nH   0.554pF
 A10   SA   CONTROL   130m   1.44nH   0.546pF
 A11   CQ   ECHO   202m   2.94nH   0.807pF
 B1   NC   NC
 B2   Q9   PROGBUF   208m   2.60nH   0.845pF
 B3   D9   DIN   225m   2.97nH   0.904pF
 B4   SA   CONTROL   189m   2.46nH   0.773pF
 B5   NC   NC
 B6   K   CONTROL   178m   2.43nH   0.753pF
 B7   NBW0   CONTROL   159m   1.94nH   0.700pF
 B8   SA   CONTROL   164m   1.96nH   0.641pF
 B9   NC   NC
 B10   NC   NC
 B11   Q8   PROGBUF   194m   2.34nH   0.805pF
 C1   NC   NC
 C2   NC   NC
 C3   D10   DIN   220m   3.32nH   0.901pF
 C4   VSS   GND
 C5   SA   CONTROL   189m   2.60nH   0.874pF
 C6   NC   NC
 C7   SA   CONTROL   204m   2.82nH   0.820pF
 C8   VSS   GND
 C9   NC   NC
 C10   Q7   PROGBUF   215m   3.12nH   0.809pF
 C11   D8   DIN   212m   2.69nH   0.808pF
 D1   NC   NC
 D2   D11   DIN   206m   2.66nH   0.823pF
 D3   Q10   PROGBUF   189m   2.60nH   0.910pF
 D4   VSS   GND
 D5   VSS   GND
 D6   VSS   GND
 D7   VSS   GND
 D8   VSS   GND
 D9   NC   NC
 D10   NC   NC
 D11   D7   DIN   192m   2.41nH   0.793pF
 E1   NC   NC
 E2   NC   NC
 E3   Q11   PROGBUF   196m   2.78nH   0.947pF
 E4   VDDQ   POWER
 E5   VSS   GND
 E6   VSS   GND
 E7   VSS   GND
 E8   VDDQ   POWER
 E9   NC   NC
 E10   D6   DIN   202m   2.76nH   0.779pF
 E11   Q6   PROGBUF   196m   2.42nH   0.803pF
 F1   NC   NC
 F2   Q12   PROGBUF   211m   2.71nH   0.850pF
 F3   D12   DIN   184m   2.63nH   0.913pF
 F4   VDDQ   POWER
 F5   VDD   POWER
 F6   VSS   GND
 F7   VDD   POWER
 F8   VDDQ   POWER
 F9   NC   NC
 F10   NC   NC
 F11   Q5   PROGBUF   192m   2.33nH   0.795pF
 G1   NC   NC
 G2   D13   DIN   210m   2.94nH   0.887pF
 G3   Q13   PROGBUF   184m   2.75nH   0.946pF
 G4   VDDQ   POWER
 G5   VDD   POWER
 G6   VSS   GND
 G7   VDD   POWER
 G8   VDDQ   POWER
 G9   NC   NC
 G10   NC   NC
 G11   D5   DIN   207m   2.66nH   0.842pF
 H1   NDoff   CONTROL   165m   1.96nH   0.637pF
 H2   VREF   POWER
 H3   VDDQ   POWER
 H4   VDDQ   POWER
 H5   VDD   POWER
 H6   VSS   GND
 H7   VDD   POWER
 H8   VDDQ   POWER
 H9   VDDQ   POWER
 H10   VREF   POWER
 H11   ZQ   NC
 J1   NC   NC
 J2   NC   NC
 J3   D14   DIN   226m   3.23nH   0.948pF
 J4   VDDQ   POWER
 J5   VDD   POWER
 J6   VSS   GND
 J7   VDD   POWER
 J8   VDDQ   POWER
 J9   NC   NC
 J10   Q4   PROGBUF   205m   2.81nH   0.844pF
 J11   D4   DIN   202m   2.51nH   0.823pF
 K1   NC   NC
 K2   NC   NC
 K3   Q14   PROGBUF   189m   2.85nH   0.951pF
 K4   VDDQ   POWER
 K5   VDD   POWER
 K6   VSS   GND
 K7   VDD   POWER
 K8   VDDQ   POWER
 K9   NC   NC
 K10   D3   DIN   202m   2.80nH   0.834pF
 K11   Q3   PROGBUF   192m   2.33nH   0.811pF
 L1   NC   NC
 L2   Q15   PROGBUF   174m   2.27nH   0.866pF
 L3   D15   DIN   185m   2.74nH   0.923pF
 L4   VDDQ   POWER
 L5   VSS   GND
 L6   VSS   GND
 L7   VSS   GND
 L8   VDDQ   POWER
 L9   NC   NC
 L10   NC   NC
 L11   Q2   PROGBUF   193m   2.31nH   0.828pF
 M1   NC   NC
 M2   NC   NC
 M3   D16   DIN   227m   3.44nH   0.929pF
 M4   VSS   GND
 M5   VSS   GND
 M6   VSS   GND
 M7   VSS   GND
 M8   VSS   GND
 M9   NC   NC
 M10   Q1   PROGBUF   208m   3.05nH   0.827pF
 M11   D2   DIN   209m   2.65nH   0.828pF
 N1   NC   NC
 N2   D17   DIN   201m   2.68nH   0.874pF
 N3   Q16   PROGBUF   186m   2.86nH   0.943pF
 N4   VSS   GND
 N5   SA   CONTROL   188m   2.45nH   0.921pF
 N6   SA   CONTROL   204m   2.83nH   0.868pF
 N7   SA   CONTROL   163m   2.11nH   0.852pF
 N8   VSS   GND
 N9   NC   NC
 N10   NC   NC
 N11   D1   DIN   190m   2.33nH   0.805pF
 P1   NC   NC
 P2   NC   NC
 P3   Q17   PROGBUF   186m   2.78nH   0.889pF
 P4   SA   CONTROL   146m   1.90nH   0.747pF
 P5   SA   CONTROL   212m   3.30nH   0.853pF
 P6   QVLD   ECHO   186m   2.56nH   0.853pF
 P7   SA   CONTROL   161m   2.06nH   0.701pF
 P8   SA   CONTROL   161m   2.05nH   0.660pF
 P9   NC   NC
 P10   D0   DIN   200m   2.92nH   0.813pF
 P11   Q0   PROGBUF   199m   2.52nH   0.815pF
 R1   TDO   JTAG   160m   2.03nH   0.671pF
 R2   TCK   CONTROL   166m   2.10nH   0.712pF
 R3   SA   CONTROL   153m   2.12nH   0.662pF
 R4   SA   CONTROL   180m   2.75nH   0.761pF
 R5   SA   CONTROL   176m   2.69nH   0.749pF
 R6   NC   NC
 R7   SA   CONTROL   177m   2.32nH   0.736pF
 R8   SA   CONTROL   137m   1.63nH   0.576pF
 R9   SA   CONTROL   125m   1.39nH   0.547pF
 R10   TMS   CONTROL   131m   1.64nH   0.560pF
 R11   TDI   CONTROL   970m   0.91nH   0.503pF
[Component]   GS81302D36E
[Manufacturer]   GSI Technology
[Package]
|  variable   typ   min   max
R_pkg   0.2   0.1   0.5
L_pkg   3nH   1nH   5nH
C_pkg   1.5pF   1pF   3pF
[Package Model]   81302xxxE
[Pin Mapping] pulldown_ref pullup_ref gnd_clamp_ref power_clamp_ref ext_ref
|PIN   Pull-Down   Pull-Up   Power-clamp   Gnd-clamp   EXT-ref
 A1   VSS   VDDQ   VSS   VDD
 A2   NC   NC
 A3   NC   NC   VSS   VDD   VREF
 A4   NC   NC   VSS   VDD   VREF
 A5   NC   NC   VSS   VDD   VREF
 A6   NC   NC   VSS   VDD   VREF
 A7   NC   NC   VSS   VDD   VREF
 A8   NC   NC   VSS   VDD   VREF
 A9   NC   NC   VSS   VDD   VREF
 A10   NC   NC   VSS   VDD   VREF
 A11   VSS   VDDQ   VSS   VDD
 B1   VSS   VDDQ   VSS   VDD
 B2   VSS   VDDQ   VSS   VDD
 B3   NC   NC   VSS   VDD   VREF
 B4   NC   NC   VSS   VDD   VREF
 B5   NC   NC   VSS   VDD   VREF
 B6   NC   NC   VSS   VDD   VREF
 B7   NC   NC   VSS   VDD   VREF
 B8   NC   NC   VSS   VDD   VREF
 B9   NC   NC   VSS   VDD   VREF
 B10   VSS   VDDQ   VSS   VDD
 B11   VSS   VDDQ   VSS   VDD
 C1   NC   NC   VSS   VDD   VREF
 C2   VSS   VDDQ   VSS   VDD
 C3   NC   NC   VSS   VDD   VREF
 C4   VSS   NC
 C5   NC   NC   VSS   VDD   VREF
 C6   NC   NC
 C7   NC   NC   VSS   VDD   VREF
 C8   VSS   NC
 C9   NC   NC   VSS   VDD   VREF
 C10   VSS   VDDQ   VSS   VDD
 C11   NC   NC   VSS   VDD   VREF
 D1   NC   NC   VSS   VDD   VREF
 D2   NC   NC   VSS   VDD   VREF
 D3   VSS   VDDQ   VSS   VDD
 D4   VSS   NC
 D5   VSS   NC
 D6   VSS   NC
 D7   VSS   NC
 D8   VSS   NC
 D9   VSS   VDDQ   VSS   VDD
 D10   NC   NC   VSS   VDD   VREF
 D11   NC   NC   VSS   VDD   VREF
 E1   VSS   VDDQ   VSS   VDD
 E2   NC   NC   VSS   VDD   VREF
 E3   VSS   VDDQ   VSS   VDD
 E4   NC   VDDQ
 E5   VSS   NC
 E6   VSS   NC
 E7   VSS   NC
 E8   NC   VDDQ
 E9   VSS   VDDQ   VSS   VDD
 E10   NC   NC   VSS   VDD   VREF
 E11   VSS   VDDQ   VSS   VDD
 F1   VSS   VDDQ   VSS   VDD
 F2   VSS   VDDQ   VSS   VDD
 F3   NC   NC   VSS   VDD   VREF
 F4   NC   VDDQ
 F5   NC   VDD
 F6   VSS   NC
 F7   NC   VDD
 F8   NC   VDDQ
 F9   NC   NC   VSS   VDD   VREF
 F10   VSS   VDDQ   VSS   VDD
 F11   VSS   VDDQ   VSS   VDD
 G1   NC   NC   VSS   VDD   VREF
 G2   NC   NC   VSS   VDD   VREF
 G3   VSS   VDDQ   VSS   VDD
 G4   NC   VDDQ
 G5   NC   VDD
 G6   VSS   NC
 G7   NC   VDD
 G8   NC   VDDQ
 G9   VSS   VDDQ   VSS   VDD
 G10   NC   NC   VSS   VDD   VREF
 G11   NC   NC   VSS   VDD   VREF
 H1   NC   NC   VSS   VDD   VREF
 H2   NC   VREF
 H3   NC   VDDQ
 H4   NC   VDDQ
 H5   NC   VDD
 H6   VSS   NC
 H7   NC   VDD
 H8   NC   VDDQ
 H9   NC   VDDQ
 H10   NC   VREF
 H11   NC   NC
 J1   NC   NC   VSS   VDD   VREF
 J2   VSS   VDDQ   VSS   VDD
 J3   NC   NC   VSS   VDD   VREF
 J4   NC   VDDQ
 J5   NC   VDD
 J6   VSS   NC
 J7   NC   VDD
 J8   NC   VDDQ
 J9   NC   NC   VSS   VDD   VREF
 J10   VSS   VDDQ   VSS   VDD
 J11   NC   NC   VSS   VDD   VREF
 K1   VSS   VDDQ   VSS   VDD
 K2   NC   NC   VSS   VDD   VREF
 K3   VSS   VDDQ   VSS   VDD
 K4   NC   VDDQ
 K5   NC   VDD
 K6   VSS   NC
 K7   NC   VDD
 K8   NC   VDDQ
 K9   VSS   VDDQ   VSS   VDD
 K10   NC   NC   VSS   VDD   VREF
 K11   VSS   VDDQ   VSS   VDD
 L1   VSS   VDDQ   VSS   VDD
 L2   VSS   VDDQ   VSS   VDD
 L3   NC   NC   VSS   VDD   VREF
 L4   NC   VDDQ
 L5   VSS   NC
 L6   VSS   NC
 L7   VSS   NC
 L8   NC   VDDQ
 L9   NC   NC   VSS   VDD   VREF
 L10   VSS   VDDQ   VSS   VDD
 L11   VSS   VDDQ   VSS   VDD
 M1   NC   NC   VSS   VDD   VREF
 M2   VSS   VDDQ   VSS   VDD
 M3   NC   NC   VSS   VDD   VREF
 M4   VSS   NC
 M5   VSS   NC
 M6   VSS   NC
 M7   VSS   NC
 M8   VSS   NC
 M9   NC   NC   VSS   VDD   VREF
 M10   VSS   VDDQ   VSS   VDD
 M11   NC   NC   VSS   VDD   VREF
 N1   NC   NC   VSS   VDD   VREF
 N2   NC   NC   VSS   VDD   VREF
 N3   VSS   VDDQ   VSS   VDD
 N4   VSS   NC
 N5   NC   NC   VSS   VDD   VREF
 N6   NC   NC   VSS   VDD   VREF
 N7   NC   NC   VSS   VDD   VREF
 N8   VSS   NC
 N9   VSS   VDDQ   VSS   VDD
 N10   NC   NC   VSS   VDD   VREF
 N11   NC   NC   VSS   VDD   VREF
 P1   VSS   VDDQ   VSS   VDD
 P2   NC   NC   VSS   VDD   VREF
 P3   VSS   VDDQ   VSS   VDD
 P4   NC   NC   VSS   VDD   VREF
 P5   NC   NC   VSS   VDD   VREF
 P6   NC   NC   VSS   VDD   VREF
 P7   NC   NC   VSS   VDD   VREF
 P8   NC   NC   VSS   VDD   VREF
 P9   VSS   VDDQ   VSS   VDD
 P10   NC   NC   VSS   VDD   VREF
 P11   VSS   VDDQ   VSS   VDD
 R1   VSS   VDDQ   VSS   VDD
 R2   NC   NC   VSS   VDD   VREF
 R3   NC   NC   VSS   VDD   VREF
 R4   NC   NC   VSS   VDD   VREF
 R5   NC   NC   VSS   VDD   VREF
 R6   NC   NC   VSS   VDD   VREF
 R7   NC   NC   VSS   VDD   VREF
 R8   NC   NC   VSS   VDD   VREF
 R9   NC   NC   VSS   VDD   VREF
 R10   NC   NC   VSS   VDD   VREF
 R11   NC   NC   VSS   VDD   VREF
[Pin]   signal_name model_name   R_pin   L_pin   C_pin
 A1   nCQ   ECHO   197m   2.83nH   0.820pF
 A2   NC   NC
 A3   SA   CONTROL   150m   1.95nH   0.604pF
 A4   nW   CONTROL   138m   1.73nH   0.628pF
 A5   nBW2   CONTROL   139m   1.69nH   0.633pF
 A6   nK   CONTROL   178m   2.50nH   0.709pF
 A7   nBW1   CONTROL   153m   1.96nH   0.651pF
 A8   nR   CONTROL   132m   1.54nH   0.560pF
 A9   SA   CONTROL   131m   1.40nH   0.554pF
 A10   SA   CONTROL   130m   1.44nH   0.546pF
 A11   CQ   ECHO   202m   2.94nH   0.807pF
 B1   Q27   PROGBUF   195m   2.39nH   0.827pF
 B2   Q18   PROGBUF   208m   2.60nH   0.845pF
 B3   D18   DIN   225m   2.97nH   0.904pF
 B4   SA   CONTROL   189m   2.46nH   0.773pF
 B5   nBW3   CONTROL   120m   1.43nH   0.622pF
 B6   K   CONTROL   178m   2.43nH   0.753pF
 B7   NBW0   CONTROL   159m   1.94nH   0.700pF
 B8   SA   CONTROL   164m   1.96nH   0.641pF
 B9   D17   DIN   188m   2.61nH   0.868pF
 B10   Q17   PROGBUF   209m   2.72nH   0.835pF
 B11   Q8   PROGBUF   194m   2.34nH   0.805pF
 C1   D27   DIN   197m   2.54nH   0.785pF
 C2   Q28   PROGBUF   213m   3.17nH   0.827pF
 C3   D19   DIN   220m   3.32nH   0.901pF
 C4   VSS   GND
 C5   SA   CONTROL   189m   2.60nH   0.874pF
 C6   NC   NC
 C7   SA   CONTROL   204m   2.82nH   0.820pF
 C8   VSS   GND
 C9   D16   DIN   224m   3.31nH   0.905pF
 C10   Q7   PROGBUF   215m   3.12nH   0.809pF
 C11   D8   DIN   212m   2.69nH   0.808pF
 D1   D28   DIN   189m   2.32nH   0.778pF
 D2   D20   DIN   206m   2.66nH   0.823pF
 D3   Q19   PROGBUF   189m   2.60nH   0.910pF
 D4   VSS   GND
 D5   VSS   GND
 D6   VSS   GND
 D7   VSS   GND
 D8   VSS   GND
 D9   Q16   PROGBUF   182m   2.62nH   0.898pF
 D10   D15   DIN   199m   2.68nH   0.830pF
 D11   D7   DIN   192m   2.41nH   0.793pF
 E1   Q29   PROGBUF   192m   2.33nH   0.813pF
 E2   D29   DIN   204m   2.70nH   0.797pF
 E3   Q20   PROGBUF   196m   2.78nH   0.947pF
 E4   VDDQ   POWER
 E5   VSS   GND
 E6   VSS   GND
 E7   VSS   GND
 E8   VDDQ   POWER
 E9   Q15   PROGBUF   183m   2.64nH   0.876pF
 E10   D6   DIN   202m   2.76nH   0.779pF
 E11   Q6   PROGBUF   196m   2.42nH   0.803pF
 F1   Q30   PROGBUF   192m   2.40nH   0.794pF
 F2   Q21   PROGBUF   211m   2.71nH   0.850pF
 F3   D21   DIN   184m   2.63nH   0.913pF
 F4   VDDQ   POWER
 F5   VDD   POWER
 F6   VSS   GND
 F7   VDD   POWER
 F8   VDDQ   POWER
 F9   D14   DIN   177m   2.82nH   0.841pF
 F10   Q14   PROGBUF   202m   2.76nH   0.833pF
 F11   Q5   PROGBUF   192m   2.33nH   0.795pF
 G1   D30   DIN   200m   2.50nH   0.814pF
 G2   D22   DIN   210m   2.94nH   0.887pF
 G3   Q22   PROGBUF   184m   2.75nH   0.946pF
 G4   VDDQ   POWER
 G5   VDD   POWER
 G6   VSS   GND
 G7   VDD   POWER
 G8   VDDQ   POWER
 G9   Q13   PROGBUF   186m   2.45nH   0.896pF
 G10   D13   DIN   209m   2.99nH   0.859pF
 G11   D5   DIN   207m   2.66nH   0.842pF
 H1   NDoff   CONTROL   165m   1.96nH   0.637pF
 H2   VREF   POWER
 H3   VDDQ   POWER
 H4   VDDQ   POWER
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| Models and submodels in the file (27): VIO_18_50 (I/O), VIO_15_50 (I/O), VIO_18_35 (I/O), VIO_15_35 (I/O), VIO_18_50_ODT (I/O), VIO_15_50_ODT (I/O), VIO_18_35_ODT (I/O), VIO_15_35_ODT (I/O), VOUT_18_50 (Output), VOUT_15_50 (Output), VOUT_18_35 (Output), VOUT_15_35 (Output), JTAG (Output), VCQ_18_50 (Output), VCQ_15_50 (Output), VCQ_18_35 (Output), VCQ_15_35 (Output), CONTROL_18 (Input), CONTROL_15 (Input), CONTROL_18_ODT (Input), CONTROL_15_ODT (Input), DIN_18 (Input), DIN_15 (Input), DIN_18_ODT (Input), DIN_15_ODT (Input), Weak_ODT_18V (Dynamic_clamp), Weak_ODT_15V (Dynamic_clamp)
